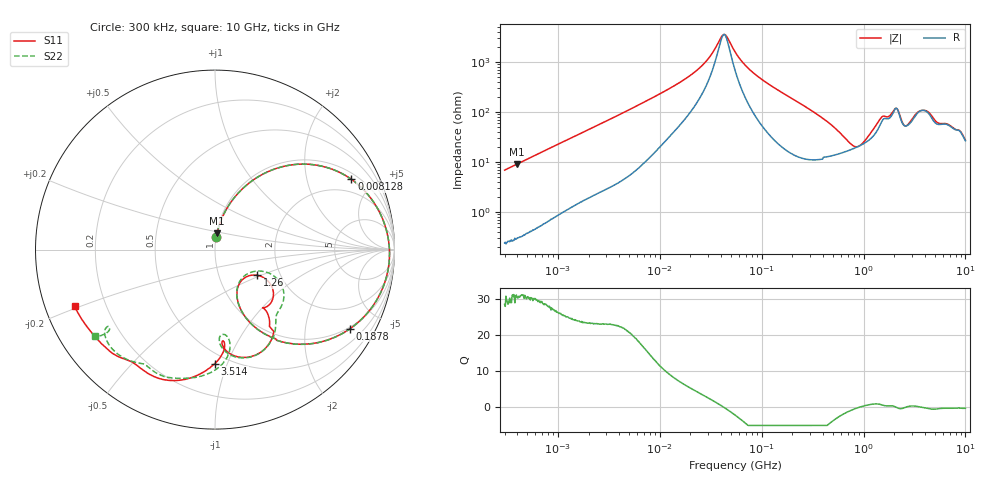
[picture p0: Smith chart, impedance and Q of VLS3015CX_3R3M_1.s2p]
! S-Parameter Data Generated by TDK Corporation
! Copyright(C) 2020 TDK Corporation.
! All Rights Reserved.
! TDK P/N: VLS3015CX-3R3M-1 (Inductor)
! Property: L=3.3uH at 1MHz
! Size(LxWxT): 3x3x1.5mm
! Model Type: s2p (Touchstone File Format Version 1.0)
! Frequency: DC=Yes Start=0.3MHz Stop=10000MHz 802points Log-sweep
! Model Generated on Aug. 18, 2020
! Port Assignments:
!  1 ---@@@--- 2
! Applicable Conditions:
!  Temperature = 25 degC
!  DC Bias Current = 0 A
!  Small Signal Operation
! Terms and conditions regarding TDK Simulation Models
! (1)This simulation model is being provided solely for informational purposes. Please refer to the specifications of the products in terms of detailed characteristics of such products.
! (2)In no event shall TDK Corporation of any of its subsidiaries be liable for any loss or damage arising, directly or indirectly,
!  From any information contained in this simulation model, including, but not limited to loss or damages arising from any inaccuracies, omissions or errors in connection with such information.
! (3)Any and all copyrights on this simulation model are owned by TDK Corporation.
!  Duplication or redistribution of this simulation model without prior written permission from TDK Corporation is prohibited.
! (4)This simulation model is subject to any modification or change without any prior notice.
! (5)Neither TDK Corporation nor any of its subsidiaries shall make any warranty, express or implied,
!  Including but not limited to the correctness, implied warranties of merchantability and fitness for a particular purpose with respect to this simulation models.
! (6)The use of this simulation model shall be deemed to have consented to the terms and conditions hereof.
# Hz S MA R 50
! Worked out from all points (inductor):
!   801 points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, 300 kHz to 10 GHz, reference 50 ohm
!   read as one part in series: L = 3.66 uH near 318.3 kHz
!   highest Q = 30.9 at 396.3 kHz (marker M1), where L = 3.66 uH
!   self-resonance near 42.75 MHz
!   S11 on the Smith chart (normalised r, x): 300 kHz: 1.00, +0.14; 8.128 MHz: 1.27, +3.71; 187.8 MHz: 0.94, -3.46; 1.26 GHz: 1.53, -0.47; 3.514 GHz: 0.42, -0.90; 10 GHz: 0.09, -0.19
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300000  0.06904 84.2  0.9952 -3.9  0.995 -3.9  0.06885 84.1
396270  0.09078 83.0  0.993 -5.2  0.9927 -5.2  0.09033 83.0
1713600  0.3534 66.9  0.9208 -20.7  0.9206 -20.7  0.3534 66.9
4001173  0.6492 46.9  0.7322 -40.5  0.7322 -40.5  0.6492 46.9
8128066  0.8549 27.3  0.4626 -58.7  0.4626 -58.7  0.8549 27.3
9671944  0.8853 23.0  0.397 -62.2  0.397 -62.2  0.8853 23.0
2.441527e7  0.9612 6.4  0.1273 -69.5  0.1273 -69.5  0.9612 6.4
4.199124e7  0.9726 -0.9  0.02756 -8.9  0.02755 -9.0  0.9727 -0.9
5.477226e7  0.9725 -4.6  0.06034 60.0  0.06034 60.0  0.9726 -4.6
8.740098e7  0.9607 -12.1  0.1714 69.5  0.1713 69.5  0.9608 -12.2
1.878293e8  0.8727 -30.3  0.4263 55.4  0.4263 55.4  0.8727 -30.3
3.126428e8  0.7163 -47.4  0.6308 36.9  0.6308 36.9  0.7164 -47.5
6.821612e8  0.3476 -66.7  0.8089 0.3  0.8088 0.3  0.3469 -66.8
1.001841e9  0.2283 -51.1  0.7943 -20.5  0.7942 -20.5  0.2227 -50.8
1.260284e9  0.276 -31.3  0.7248 -35.8  0.7248 -35.9  0.2626 -27.1
1.767019e9  0.4215 -50.5  0.5238 -46.2  0.524 -46.2  0.5018 -47.1
2.08171e9  0.5959 -58.5  0.3897 -45.5  0.3899 -45.6  0.6167 -62.5
2.507534e9  0.5535 -84.6  0.5232 -41.8  0.5231 -41.9  0.5223 -87.1
3.514172e9  0.6356 -90.1  0.3401 -71.2  0.3397 -71.2  0.6599 -88.6
4.632637e9  0.7806 -112.6  0.2771 -62.3  0.2768 -62.3  0.7599 -111.2
8.322921e9  0.8246 -143.1  0.1948 -88.6  0.1947 -88.6  0.7378 -144.4
1e10  0.8434 -157.9  0.1927 -88.0  0.1926 -88.0  0.8251 -144.1
